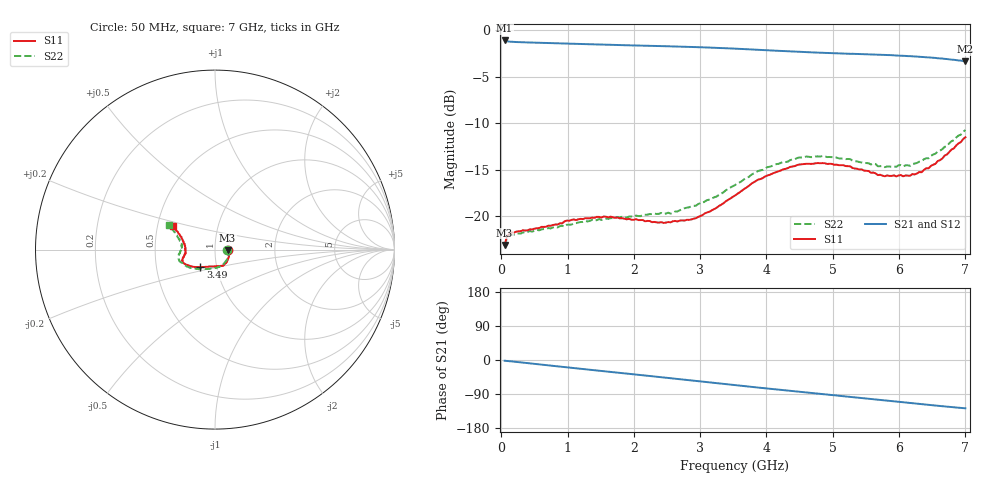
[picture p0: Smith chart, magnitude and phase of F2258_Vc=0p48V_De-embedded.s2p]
! Integrated Device Technology
! Corporate Headquarters
! 6024 Silver Creek Valley Road
! San Jose, CA 95138  USA
! Phone:  1-408-284-8200
! Toll Free:  1-800-223-1366
! Webpage:  http://www.idt.com/
! Timing and RF Division
! 515 Groton Road, Suite 102
! Westford, MA 01886-6024
! Device:  F2258
! Description: Voltage Variable RF Attenuator
! Frequency:  50.0 -  6000.00 MHz
! Package:  3x3 mm Thin QFN Plastic Package: 16 pin
! Ports:  2 RF, 2 DC
!  Pin  1  = NC
!  Pin  2  = NC
!  Pin  3  = RF2  = Port 2
!  Pin  4  = GND
!  Pin  5  = Vdd
!  Pin  6  = NC
!  Pin  7  = VCTRL
!  Pin  8  = NC
!  Pin  9  = GND
!  Pin 10  = RF1  = Port 1
!  Pin 11  = NC
!  Pin 12  = NC
!  Pin 13  = NC
!  Pin 14  = NC
!  Pin 15  = NC
!  Pin 16  = NC
! Vcntrl:  0.480 Volts
! Vdd:  +3.300 Volts
! Current:  1.099 mA
! Data:  The device was measured on a the F2258 evaluation board which has
!  individual transmission lines to the RF pins.  Data was collected
!  using a calibrated network analyzer.  The evaluation board was
!  de-embedded using a TRL calibration technique.
!  The reference plane is the edge of the package pin.
! Misc:  SN 10
!  Action Tracker AT0285
! Date Measured:  2014-12-10
! Date:  2016-01-13  MJV
! Note:
!  Integrated Device Technology supplies this data as a sample of measured
!  data at the package pin for this product.  Your particular data for this
!  product may vary.
!  Data was taken at 25 degrees C.
!  Integrated Device Technology reserves the right to change this data at anytime.
!Freq_(GHz)  S11M_(dB)  S11P_(deg)  S21M_(dB)  S21P_(deg)  S12M_(dB)  S12P_(deg)  S22M_(dB)  S22P_(deg)
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# GHz S dB R 50
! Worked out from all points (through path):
!   201 points, 50 MHz to 7 GHz, reference 50 ohm
!   highest |S21| = -1.08 dB at 50 MHz (marker M1); lowest = -3.3 dB at 7 GHz (marker M2)
!   group delay of S21, straight-line fit = 50.5 ps
!   lowest |S11| = -23.1 dB at 50 MHz (marker M3), VSWR 1.15, Z = 57.5 - j0.443 ohm
!   |S11| at or under -10 dB: start of sweep to end of sweep
!   |S22| runs from -23.2 to -10.7 dB; largest |S21 - S12| = 0.00038
!   S11 on the Smith chart (normalised r, x): 50 MHz: 1.15, -0.01; 3.49 GHz: 0.83, -0.16; 7 GHz: 0.61, +0.17
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0.05  -23.12 -3.1  -1.08 -2.0  -1.08 -2.0  -23.24 -3.1
0.08475  -22.20 -5.1  -1.17 -2.5  -1.17 -2.5  -22.34 -5.0
0.15425  -21.75 -7.9  -1.22 -3.7  -1.22 -3.7  -21.99 -8.7
0.71025  -21.03 -32.6  -1.36 -14.1  -1.36 -14.1  -21.29 -35.8
1.2315  -20.32 -53.1  -1.47 -23.8  -1.47 -23.8  -20.63 -59.7
1.6485  -20.05 -64.3  -1.55 -31.4  -1.55 -31.4  -20.22 -72.9
2.37825  -20.70 -84.0  -1.68 -44.8  -1.68 -44.8  -19.75 -91.2
2.552  -20.67 -89.7  -1.72 -48.0  -1.72 -48.0  -19.73 -96.6
2.93425  -20.22 -106.3  -1.80 -55.1  -1.80 -55.1  -18.88 -110.2
3.247  -19.10 -119.9  -1.87 -61.0  -1.87 -61.0  -17.89 -122.5
3.49025  -17.93 -130.2  -1.95 -65.6  -1.95 -65.6  -16.79 -131.8
3.525  -17.78 -131.2  -1.96 -66.2  -1.96 -66.2  -16.66 -133.3
4.0115  -15.62 -146.4  -2.14 -75.3  -2.14 -75.3  -14.73 -149.2
4.46325  -14.49 -155.5  -2.30 -83.4  -2.30 -83.4  -13.74 -160.5
4.7065  -14.36 -158.8  -2.37 -87.7  -2.37 -87.7  -13.63 -164.9
5.2625  -14.63 -165.5  -2.52 -97.4  -2.52 -97.4  -13.86 -173.2
5.6795  -15.58 -171.9  -2.61 -104.6  -2.61 -104.6  -14.63 -178.8
5.85325  -15.67 -176.1  -2.66 -107.8  -2.66 -107.8  -14.66 176.5
6.166  -15.65 175.9  -2.77 -113.4  -2.77 -113.3  -14.58 170.5
6.33975  -15.28 169.2  -2.85 -116.4  -2.85 -116.4  -14.08 166.0
6.722  -13.36 156.6  -3.08 -123.1  -3.08 -123.1  -12.45 156.9
7  -11.51 150.5  -3.33 -127.4  -3.33 -127.4  -10.73 151.8
